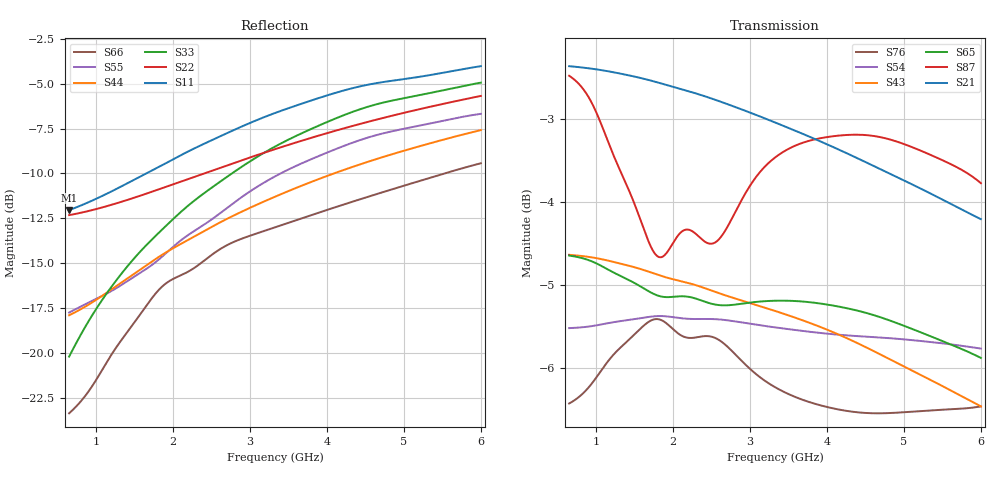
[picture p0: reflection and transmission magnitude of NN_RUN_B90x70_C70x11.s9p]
! IGNION VIRTUAL ANTENNA LIBRARY
! NN_RUN_B90x70_C70x11
! Virtual Antenna™ RUN mXTEND™: NN02-224 12.0 mm x 3.0 mm x 2.4 mm
! https://ignion.io/product/run-mxtend/
! Board: 90 mm x 70 mm
! Clearance Area: 70 mm x 11 mm
! Feeding line: L-shape; 11mm x 2mm and 5mm x 2mm
! Applications: Fleet management, IoT
! Frequency range 0.65GHz to 6GHz, step 10MHz
! Number of ports 9
! This product and its use is protected by at least one or more of the following patents and patent
! applications US 8,203,492 B2; US 8,237,615 B2; PCT/EP2013/064692; WO 2014/012842 A1; US 2019/190122 A1;
! US 62/072,671; and other domestic and international patents pending. Additional information about
! patents related to this product is available at https://ignion.io/files/Patent-list-NN.pdf, all
! rights reserved. Copyright, Ignion 2021.
! Need more help? Your platform is much different than these examples in the manual? Use our
! Fast Track service (https://ignion.io/fast-track/), for free, and get a personalized antenna design in
! just 24 hours.
! Touchstone port 1 = "Series Port"
! Touchstone port 2 = "Shunt Port"
! Touchstone port 3 = "Series Port"
! Touchstone port 4 = "Shunt Port"
! Touchstone port 5 = "Series Port"
! Touchstone port 6 = "Shunt Port"
! Touchstone port 7 = "Series Port"
! Touchstone port 8 = "Shunt Port"
! Touchstone port 9 = "Series Port"
! IE3D S-Parameters Output Version 2.0
# GHZ S MA R 50
! Nport = 9
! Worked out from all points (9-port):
!   536 points, 650 MHz to 6 GHz, reference 50 ohm
!   strongest paths, dB at 650 MHz, 1.99 GHz, 3.33 GHz, 4.67 GHz, 6 GHz:
!     S21: -2.4, -2.6, -3.0, -3.6, -4.2
!     S87: -2.5, -4.5, -3.5, -3.2, -3.8
!     S65: -4.6, -5.1, -5.2, -5.4, -5.9
!     S43: -4.6, -4.9, -5.3, -5.8, -6.5
!     S54: -5.5, -5.4, -5.5, -5.6, -5.8
!     S76: -6.4, -5.5, -6.2, -6.5, -6.5
!   lowest |S11| = -12.0 dB at 650 MHz (marker M1), VSWR 1.67, Z = 31.1 + j7.72 ohm
!   |S11| at or under -10 dB: start of sweep to 1.655 GHz
